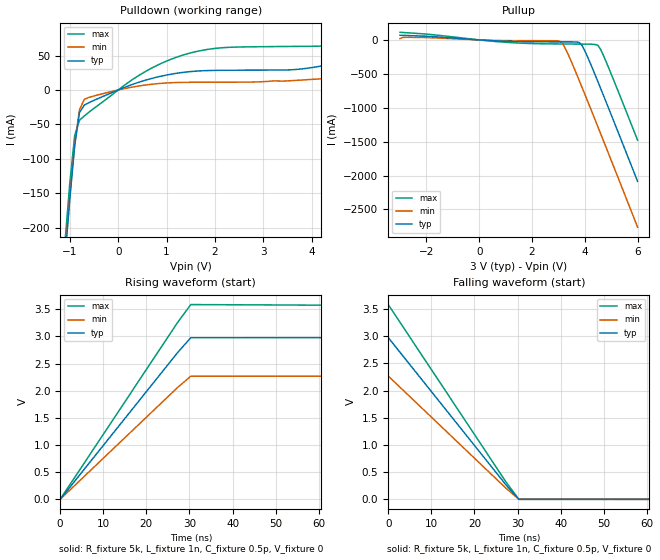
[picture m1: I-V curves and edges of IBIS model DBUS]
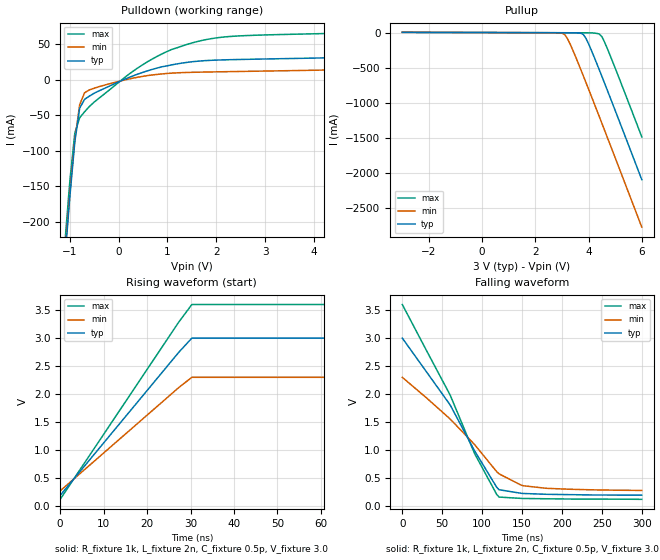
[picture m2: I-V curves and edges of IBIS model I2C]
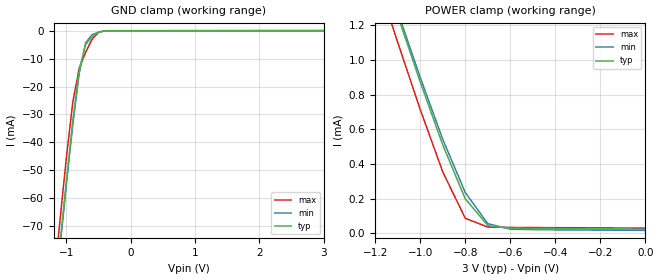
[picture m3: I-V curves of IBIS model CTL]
| Philips Semiconductors Inc.
| Specialty Products Group
| IBIS model of PCA9564
| Parallel bus to I2C-bus controller
| 20-pin SO, TSSOP and HVQFN Packages
[IBIS Ver]   3.2
[Comment Char]   |_char
[File name]   pca9564.ibs
[File Rev]   1.0
[Date]   Aug 4, 2003 10:50:08 AM
[Source]   Generated with Ibis Toolkit
[Notes]   Generated by TGA
[Copyright]  2003 Philips Semiconductors
[Disclaimer]
* All rights reserved
Philips Semiconductors warrants and represents that the SPICE models
identified herein are owned by Philips Semiconductors (PHILIPS).  The
models provided are not warranted as fully representing all of the
operating characteristics and specifications of the semiconductor
products to which the models relate.  Moreover, unless there is a
signed, written agreement to the contrary, these models are furnished
on an "as is" basis without support or warranty of any kind, either
expressed or implied, regarding the use thereof, and PHILIPS
specifically disclaims all implied warranties of merchantability and
fitness of the models for any purpose.
PHILIPS does not assume any liability arising out of the application
or use of these SPICE models including infringement of patents and
copyrights, nor does PHILIPS convey any license under its patents and
copyrights or the rights of others.
PHILIPS provides SPICE models as a service to our customers.  You and
your company shall not distribute, convey, sell, or give these models
to anyone else without receiving prior written permission from
PHILIPS.
[Component]   PCA9564D
Si_location Pin
Timing_location Pin
[Manufacturer]   Philips Semiconductors
| [Package]   SO20
[Package]
| variable   typ   min   max
R_pkg   5.95E-02   5.36E-02   6.59E-02
L_pkg   4.21E-09   3.07E-09   5.91E-09
C_pkg   0.910E-12  0.758E-12  1.110E-12
[Pin] signal_name   model_name   R_pin	  L_pin   C_pin
1   D0   DBUS   6.63E-02  3.18E-09  0.408E-12
2   D1   DBUS   6.67E-02  2.55E-09  0.398E-12
3   D2   DBUS   8.34E-02  2.35E-09  0.317E-12
4   D3   DBUS   7.44E-02  2.16E-09  0.293E-12
5   D4   DBUS   7.10E-02  2.09E-09  0.282E-12
6   D5   DBUS   7.10E-02  2.09E-09  0.282E-12
7   D6   DBUS   7.44E-02  2.16E-09  0.293E-12
8   D7   DBUS   8.34E-02  2.35E-09  0.317E-12
9   NC   NC   6.67E-02  2.55E-09  0.397E-12
10   Vss   GND   6.63E-02  3.18E-09  0.420E-12
11   WRn   CTL   6.63E-02  3.17E-09  0.420E-12
12   RDn   CTL   6.67E-02  2.55E-09  0.397E-12
13   CEn   CTL   8.34E-02  2.35E-09  0.317E-12
14   A0   CTL   7.44E-02  2.16E-09  0.293E-12
15   A1   CTL   7.10E-02  2.09E-09  0.282E-12
16   INTn   INT   7.10E-02  2.09E-09  0.282E-12
17   RESETn   CTL   7.44E-02  2.16E-09  0.293E-12
18   SCL   I2C   8.34E-02  2.35E-09  0.317E-12
19   SDA   I2C   6.67E-02  2.55E-09  0.398E-12
20   Vdd   POWER   6.63E-02  3.17E-09  0.420E-12
[Component]   PCA9564PW
[Manufacturer]   Philips Semiconductors
[Package]
| [Package]   TSSOP20
| variable   typ   min   max
R_pkg   7.24E-02   6.63E-02   8.34E-02
L_pkg   2.47E-09   2.09E-09   3.18E-09
C_pkg   0.341E-12  0.282E-12  0.420E-12
| SO20
[Pin] signal_name   model_name   R_pin   L_pin   C_pin
1   D0   DBUS   6.63E-02  3.18E-09  0.408E-12
2   D1   DBUS   6.67E-02  2.55E-09  0.398E-12
3   D2   DBUS   8.34E-02  2.35E-09  0.317E-12
4   D3   DBUS   7.44E-02  2.16E-09  0.293E-12
5   D4   DBUS   7.10E-02  2.09E-09  0.282E-12
6   D5   DBUS   7.10E-02  2.09E-09  0.282E-12
7   D6   DBUS   7.44E-02  2.16E-09  0.293E-12
8   D7   DBUS   8.34E-02  2.35E-09  0.317E-12
9   NC   NC   6.67E-02  2.55E-09  0.397E-12
10   Vss   GND   6.63E-02  3.18E-09  0.420E-12
11   WRn   CTL   6.63E-02  3.17E-09  0.420E-12
12   RDn   CTL   6.67E-02  2.55E-09  0.397E-12
13   CEn   CTL   8.34E-02  2.35E-09  0.317E-12
14   A0   CTL   7.44E-02  2.16E-09  0.293E-12
15   A1   CTL   7.10E-02  2.09E-09  0.282E-12
16   INTn   INT   7.10E-02  2.09E-09  0.282E-12
17   RESETn   CTL   7.44E-02  2.16E-09  0.293E-12
18   SCL   I2C   8.34E-02  2.35E-09  0.317E-12
19   SDA   I2C   6.67E-02  2.55E-09  0.398E-12
20   Vdd   POWER   6.63E-02  3.17E-09  0.420E-12
[Component]   PCA9564BS
[Manufacturer]   Philips Semiconductors
[Package]
| [Package]   HVQFN20
R_pkg   0.364   0.215   0.513
L_pkg   1.486n   1.035n   1.937n
C_pkg   0.149p   0.124p   0.173p
[Package Model]  hvqfn20
[Pin] signal_name   model_name
1   D2   DBUS
2   D3   DBUS
3   D4   DBUS
4   D5   DBUS
5   D6   DBUS
6   D7   DBUS
7   NC   NC
8   Vss   GND
9   WRn   CTL
10   RDn   CTL
11   CEn   CTL
12   A0   CTL
13   A1   CTL
14   INTn   INT
15   RESETn   CTL
16   SCL   I2C
17   SDA   I2C
18   Vdd   POWER
19   D0   DBUS
20   D1   DBUS
| Models and submodels in the file (4): DBUS (Output), I2C (Output), CTL (Input), INT (Output)
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[Model]   DBUS
Model_type Output
C_comp   0.5p   0.5p   0.5p
[Temperature Range] 27   85   -40
[Voltage Range]   3   2.3   3.6
[Pullup Reference]  3   2.3   3.6
[Pulldown Reference]0   0   0
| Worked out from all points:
|   slope of the pulldown table from 0 to 0.45 V, typ, clamps not added: 38.3 ohm
|   slope of the pullup table from 0 to 0.45 V, typ, clamps not added: 43.1 ohm
|   falling waveform, R_fixture 5k, L_fixture 1n, C_fixture 0.5p, V_fixture 0: 20-80 % time 18ns typ, 18ns min, 18ns max; typ from 2.98 V to 0 V
|   rising waveform, R_fixture 5k, L_fixture 1n, C_fixture 0.5p, V_fixture 0: 20-80 % time 18ns typ, 18ns min, 17.9ns max; typ from 0 V to 2.98 V
[Pullup]
-3V       68.88mA    19.52mA    111.9mA
-2.2V     56.99mA    36.72mA    91.51mA
900mV     -18.31mA   -9.364mA   -31.99mA
3.1V      -28.69mA   -29.22mA   -59.83mA
3.3V      -28.86mA   -154.7mA   -60.39mA
3.8V      -39.95mA   -609mA     -61.48mA
3.9V      -84.31mA   -704.3mA   -61.67mA
4V        -159.6mA   -800.2mA   -61.84mA
4.5V      -618.8mA   -1.285A    -80.72mA
4.6V      -714.8mA   -1.383A    -140.3mA
4.8V      -908.3mA   -1.579A    -314.3mA
6V        -2.086A    -2.761A    -1.479A
[Pulldown]
-3V       -2.086A    -2.07A     -2.071A
-1.1V     -244.5mA   -239.3mA   -221mA
-1V       -157.8mA   -154.4mA   -135mA
-900mV    -80.9mA    -79.09mA   -66.3mA
-800mV    -32.64mA   -28.41mA   -43.84mA
-600mV    -18.26mA   -10.66mA   -31.97mA
600mV     14.94mA    7.535mA    28.28mA
1.6V      27.31mA    11.19mA    55.58mA
4.3V      36.01mA    16.69mA    64.45mA
5.6V      38.8mA     23.26mA    89.64mA
5.7V      39.53mA    23.84mA    73.07mA
6V        41.94mA    25.65mA    76.74mA
[Falling Waveform]
R_fixture=5k
L_fixture=1n
C_fixture=0.5p
V_fixture=0
V_fixture_min=0
V_fixture_max=0
0s        2.976V     2.268V     3.582V
27.27ns   270.7mV    208mV      325.5mV
30.3ns    199.4uV    1.992mV    -130.4uV
300ns     109.6uV    148uV      -119.5uV
[Rising Waveform]
R_fixture=5k
L_fixture=1n
C_fixture=0.5p
V_fixture=0
V_fixture_min=0
V_fixture_max=0
0s        0V         0V         0V
27.27ns   2.706V     2.062V     3.261V
30.3ns    2.976V     2.268V     3.587V
300ns     2.978V     2.269V     3.575V
[Ramp]
R_load=5k
dV/dt_r   1.765E+0/4.335E-10   1.333E+0/7.638E-10   2.138E+0/2.635E-10
dV/dt_f   1.768E+0/8.219E-10   1.303E+0/9.475E-10   2.139E+0/7.725E-10
|[End   DBUS
[Model]   I2C
Model_type Output
C_comp   0.5p   0.5p   0.5p
[Temperature Range] 27   85   -40
[Voltage Range]   3.0   2.3   3.6
[Pullup Reference]  3.0   2.3   3.6
[Pulldown Reference]0   0   0
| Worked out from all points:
|   slope of the pulldown table from 0 to 0.45 V, typ, clamps not added: 36.4 ohm
|   slope of the pullup table from 0 to 0.45 V, typ, clamps not added: 999 ohm
|   falling waveform, R_fixture 1k, L_fixture 2n, C_fixture 0.5p, V_fixture 3.0: 20-80 % time 72.2ns typ, 81.1ns min, 69.6ns max; typ from 3 V to 0.197 V
|   rising waveform, R_fixture 1k, L_fixture 2n, C_fixture 0.5p, V_fixture 3.0: 20-80 % time 18ns typ, 18ns min, 18ns max; typ from 0.191 V to 3 V
[Pullup]
-3V       3.003mA    3.001mA    3.004mA
2.7V      -2.7mA     -2.758mA   -2.7mA
3V        -3mA       -8.134mA   -3mA
3.1V      -3.1mA     -27.96mA   -3.1mA
3.3V      -3.301mA   -157.8mA   -3.3mA
3.7V      -9.04mA    -518.2mA   -3.7mA
3.8V      -26.04mA   -612.9mA   -3.8mA
4V        -160.4mA   -804.4mA   -4.025mA
4.4V      -527.1mA   -1.192A    -19.46mA
4.5V      -622.6mA   -1.29A     -58.07mA
4.9V      -1.01A     -1.682A    -409.8mA
6V        -2.092A    -2.767A    -1.484A
[Pulldown]
-3V       -2.092A    -2.076A    -2.078A
-1.1V     -249.8mA   -244.3mA   -226.9mA
-1V       -163.5mA   -159.7mA   -141.6mA
-900mV    -87.53mA   -85.27mA   -75.18mA
-800mV    -40.04mA   -35.09mA   -53.47mA
-700mV    -27.58mA   -18.3mA    -45.1mA
-600mV    -22.93mA   -14.27mA   -37.58mA
600mV     12.75mA    5.936mA    25.69mA
1.6V      25.99mA    10.61mA    53.57mA
2.4V      28.41mA    11.57mA    61.41mA
5.2V      32.73mA    15.32mA    67.33mA
6V        35.85mA    26.05mA    71.93mA
[Falling Waveform]
R_fixture=1k
L_fixture=2n
C_fixture=0.5p
V_fixture=3.0
V_fixture_min=2.3
V_fixture_max=3.6
0s        3V         2.3V       3.6V
60.61ns   1.79V      1.547V     1.962V
90.91ns   979.9mV    1.093V     931.2mV
118.2ns   339.8mV    618.1mV    212.4mV
121.2ns   294.3mV    577.6mV    163.4mV
151.5ns   227.3mV    365.7mV    138.3mV
178.8ns   213.7mV    322mV      133.2mV
209.1ns   206.7mV    303.3mV    128.3mV
300ns     197.1mV    281.6mV    122.9mV
[Rising Waveform]
R_fixture=1k
L_fixture=2n
C_fixture=0.5p
V_fixture=3.0
V_fixture_min=2.3
V_fixture_max=3.6
0s        190.8mV    272mV      121mV
27.27ns   2.745V     2.116V     3.284V
30.3ns    3V         2.3V       3.6V
300ns     3V         2.3V       3.6V
[Ramp]
R_load=1k
dV/dt_r   8.459E-1/1.802E-8   6.137E-1/1.801E-8   1.043E+0/1.798E-8
dV/dt_f   1.683E+0/7.520E-8   1.211E+0/7.673E-8   2.085E+0/6.889E-8
|[End   I2C
[Model]   CTL
Model_type Input
Vinh=2.0
Vinl=0.8
C_comp   0.5p   0.5p   0.5p
[Temperature Range] 27   85   -40
[Voltage Range]   3   2.3   3.6
[Pullup Reference]  3   2.3   3.6
[Pulldown Reference]0   0   0
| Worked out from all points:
|   GND clamp passes 1 mA (typ) near -0.53 V on its own axis
|   POWER clamp passes 1 mA (typ) near -1.03 V on its own axis
[GND Clamp]
-3V       -557.3mA   -556.1mA   -550.3mA
-1.2V     -100.5mA   -101.3mA   -91.81mA
-1.1V     -76.76mA   -77.84mA   -68.11mA
-1V       -53.76mA   -55.1mA    -45.46mA
-900mV    -32.16mA   -33.68mA   -25.47mA
-800mV    -14.08mA   -15.28mA   -13.36mA
-700mV    -4.863mA   -4.266mA   -7.694mA
-600mV    -2.181mA   -1.401mA   -3.039mA
-500mV    -480.9uA   -540.7uA   -552.8uA
-400mV    -37.79uA   -59.57uA   -28.44uA
3V        24.3uA     56.01uA    29.04uA
[POWER Clamp]
-3V       9.127mA    9.108mA    9.009mA
-1.2V     1.653mA    1.669mA    1.501mA
-1.1V     1.258mA    1.279mA    1.102mA
-1V       873.9uA    899.9uA    714.8uA
-900mV    510.4uA    543.1uA    354.4uA
-800mV    199.7uA    235.4uA    86.87uA
-700mV    44.87uA    55.98uA    36.34uA
-600mV    29.54uA    24.19uA    34.35uA
0V        24.3uA     17.28uA    30.3uA
